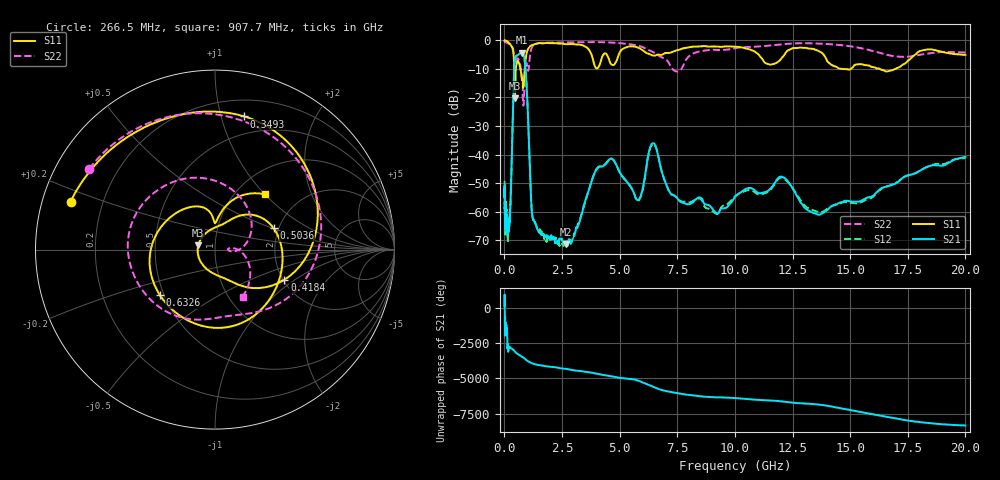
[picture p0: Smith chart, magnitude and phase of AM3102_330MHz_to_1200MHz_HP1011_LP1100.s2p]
! Date/Time: Tue, Sep 11, 2018 5:20 PM
! Network Analyzer: Agilent Technologies E8362B Rev: A.07.50.63
! Sweep from 0.010 to 20.000 GHz, 1601 Points, Sweep Type: LOG
! Power Supply: 4.949 V, 0.001 A
# Hz S DB R 50
!freq MagS11 AngS11 MagS21 AngS21 MagS12 AngS12 MagS22 AngS22
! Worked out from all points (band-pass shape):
!   1601 points, 10 MHz to 20 GHz, reference 50 ohm
!   highest |S21| = -4.30 dB at 761.4 MHz (marker M1); lowest = -71.4 dB at 2.656 GHz (marker M2)
!   |S21| within 3 dB of the highest: 447.6 MHz to 884.8 MHz (437.2 MHz wide, 65.6 % of centre)
!   lowest |S11| = -20.3 dB at 455.8 MHz (marker M3), VSWR 1.21, Z = 41.4 + j2.08 ohm
!   |S11| at or under -10 dB: 694.9 MHz to 881.5 MHz (186.6 MHz wide, 23.7 % of centre); 14.66 GHz to 15.02 GHz (357.5 MHz wide, 2.41 % of centre); 16.29 GHz to 16.96 GHz (672.1 MHz wide, 4.04 % of centre)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
!   |S22| runs from -22.9 to -0.2 dB; largest |S21 - S12| = 0.0097
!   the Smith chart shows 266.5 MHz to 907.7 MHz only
!   S11 on the Smith chart (normalised r, x): 266.5 MHz: 0.08, +0.16; 349.3 MHz: 0.34, +1.19; 418.4 MHz: 2.03, -0.83; 503.6 MHz: 1.88, +0.51; 632.6 MHz: 0.47, -0.28; 907.7 MHz: 1.35, +1.00
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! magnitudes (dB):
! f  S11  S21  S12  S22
! 10 MHz  0.0  -54.9  -49.6  -0.2
! 35.55 MHz  0.0  -64.4  -63.8  -0.5
! 126.4 MHz  -0.4  -67.5  -63.3  -0.9
! 266.5 MHz  -1.4  -56.4  -56.8  -1.6
! 349.3 MHz  -2.4  -32.1  -32.2  -2.8
! 418.4 MHz  -7.5  -11.8  -11.8  -6.0
! 447.2 MHz  -19.6  -7.3  -7.4  -8.2
! 455.8 MHz  -20.3  -6.7  -6.7  -8.4
! 503.6 MHz  -9.2  -5.5  -5.5  -7.2
! 632.6 MHz  -8.0  -4.7  -4.8  -6.9
! 761.4 MHz  -13.4  -4.3  -4.4  -13.9
! 907.7 MHz  -7.6  -9.1  -9.1  -10.3
! 1.201 GHz  -1.6  -60.7  -61.1  -2.3
! 1.59 GHz  -1.0  -67.9  -67.0  -0.9
! 2.656 GHz  -1.3  -71.4  -71.7  -0.7
! 4.112 GHz  -9.0  -44.3  -44.1  -0.6
! 5.652 GHz  -2.2  -54.3  -54.2  -1.6
! 6.457 GHz  -5.3  -36.0  -36.3  -4.1
! 7.771 GHz  -2.8  -57.0  -56.5  -8.6
! 12.03 GHz  -6.2  -47.8  -48.1  -1.4
! 13.61 GHz  -3.7  -61.1  -60.1  -1.1
! 20 GHz  -5.0  -40.8  -41.3  -4.2
